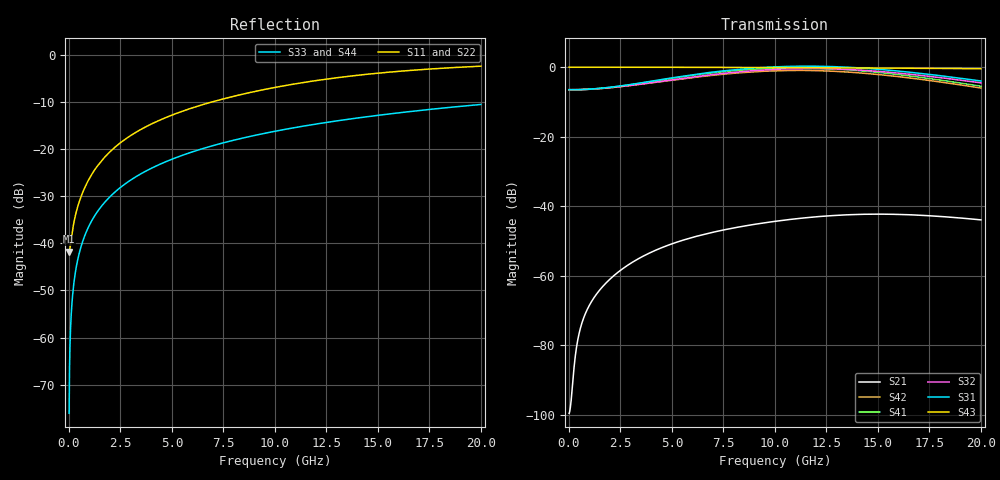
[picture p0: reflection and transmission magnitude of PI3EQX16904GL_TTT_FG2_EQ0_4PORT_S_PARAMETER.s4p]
! NPort=4 DATA=2000 NOISE=0 GROUPDELAY=0 COMPLEX_DATAFORMAT=POLAR
! NumOfBlock=1 NumOfParam=0
! .MODEL Smodel S TSTONEFILE=PI3EQX16904GL_TTT_FG2_EQ0_4PORT_S_PARAMETER.s4p TYPE=S
!  -- The above .MODEL line can be used for the S element in the netlist.
! The s parameter is extracted from the linear redriver, it is not bi-directional; only s(4,1)s(4,2) and s(3,1)s(3,2)
! should be the insertion loss
!Port definition:
!Port1 = input+
!Port2 = input-
!Port3 = output+
!Port4 = output-
# Hz S MA R  50
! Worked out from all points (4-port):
!   2000 points, 10 MHz to 20 GHz, reference 50 ohm
!   strongest paths, dB at 10 MHz, 5.01 GHz, 10.01 GHz, 15.01 GHz, 20 GHz:
!     S43: 0.0, 0.0, -0.1, -0.3, -0.4
!     S31: -6.5, -3.1, 0.1, -0.6, -4.0
!     S32: -6.5, -3.6, -0.6, -1.2, -4.5
!     S41: -6.5, -3.2, -0.3, -1.5, -5.5
!     S42: -6.5, -3.7, -1.0, -2.1, -6.0
!     S21: -99.6, -50.8, -44.3, -42.3, -43.9
!   lowest |S11| = -41.7 dB at 10 MHz (marker M1), VSWR 1.02, Z = 49.2 - j0.0603 ohm
!   |S11| at or under -10 dB: start of sweep to 6.916 GHz
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1e7  0.008182 -175.7  1.049e-05 7.4  0 0.0  0 0.0
     1.049e-05 7.4  0.008182 -175.7  0 0.0  0 0.0
     0.4742 -0.1  0.4742 179.9  0.0001571 -90.0  1 -0.0
     0.4742 179.9  0.4742 -0.1  1 -0.0  0.0001571 -90.0
2e8  0.01483 -130.6  3.318e-05 105.3  0 0.0  0 0.0
     3.318e-05 105.3  0.01483 -130.6  0 0.0  0 0.0
     0.474 -0.6  0.4739 179.2  0.003142 -90.2  1 -0.2
     0.474 179.1  0.4739 -1.1  1 -0.2  0.003142 -90.2
6.2e8  0.03268 -112.4  0.0002037 112.8  0 0.0  0 0.0
       0.0002037 112.8  0.03268 -112.4  0 0.0  0 0.0
       0.4767 -1.5  0.4759 177.8  0.009738 -90.6  0.9999 -0.6
       0.4766 177.4  0.4758 -3.3  0.9999 -0.6  0.009738 -90.6
2.97e9  0.1383 -101.7  0.00149 92.5  0 0.0  0 0.0
        0.001491 92.5  0.1383 -101.7  0 0.0  0 0.0
        0.5619 -10.7  0.5462 166.7  0.0466 -92.8  0.9988 -2.7
        0.5594 164.0  0.5437 -18.6  0.9988 -2.7  0.0466 -92.8
1.06e10  0.478 -114.5  0.00641 29.7  0 0.0  0 0.0
         0.006381 29.7  0.4769 -114.6  0 0.0  0 0.0
         1.025 -101.5  0.9459 78.6  0.1641 -99.8  0.9854 -9.4
         0.9706 60.1  0.8957 -119.7  0.9854 -9.4  0.1641 -99.8
1.475e10  0.6335 -124.4  0.007687 -6.0  0 0.0  0 0.0
          0.007683 -6.0  0.6315 -124.4  0 0.0  0 0.0
          0.9464 -164.4  0.8821 16.5  0.2252 -103.5  0.9722 -13.0
          0.8557 -9.2  0.7975 171.7  0.9722 -13.0  0.2252 -103.5
2e10  0.7613 -135.4  0.006365 -42.3  0 0.0  0 0.0
      0.006363 -42.8  0.7597 -135.3  0 0.0  0 0.0
      0.6325 125.1  0.5954 -53.8  0.2986 -108.1  0.9506 -17.4
      0.5326 -86.8  0.5013 94.3  0.9506 -17.4  0.2986 -108.1
